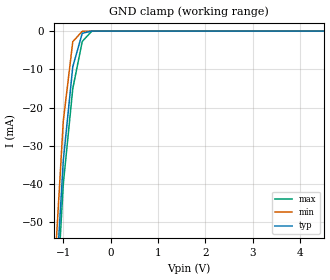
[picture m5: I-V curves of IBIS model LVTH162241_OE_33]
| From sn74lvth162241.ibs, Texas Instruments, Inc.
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|   Model LVTH162241 Input_OE_33
[Model]   LVTH162241_OE_33
Model_type  Input
Polarity   Non-Inverting
Vinl = 0.8V
Vinh = 2.0V
| variable   typ   min   max
C_comp   4pf   NA   NA
[Temperature Range]   40   -25   100
| Ambient temperature   25   -40   85
[Voltage range]   3.3   3.0   3.6
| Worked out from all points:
|   GND clamp passes 1 mA (typ) near -0.61 V on its own axis
[GND Clamp]
|   Voltage   I(typ)   I(min)   I(max)
-5V       -1.559A    -1.697A    -1.416A
-1.2V     -75.81mA   -66.12mA   -83.85mA
-1V       -33.85mA   -23.52mA   -40.01mA
-800mV    -9.342mA   -2.78mA    -15.06mA
-600mV    -586.1uA   -50.6uA    -2.71mA
-400mV    -1.379uA   -390.6nA   -54.58uA
5V        -162.1pA   81.47nA    340.7pA
